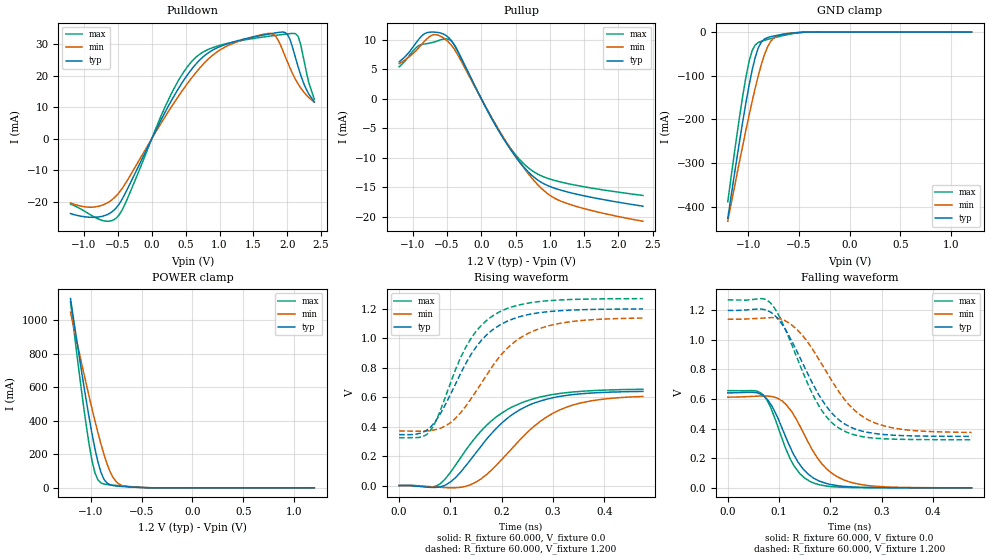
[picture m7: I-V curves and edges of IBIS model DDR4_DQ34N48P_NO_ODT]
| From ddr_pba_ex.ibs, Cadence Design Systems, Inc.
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|   Model DDR4_DQ34N48P_NO_ODT
[Model]   DDR4_DQ34N48P_NO_ODT
Model_type I/O
Polarity   Non-Inverting
Enable   Active-High
Vinl =  0.823V
Vinh =  0.887V
C_comp   1.689pF   1.691pF   1.711pF
C_comp_pullup   0.525pF   0.576pF   0.518pF
C_comp_pulldown   1.164pF   1.114pF   1.192pF
[Model Spec]
Vinh   0.887V   NA   NA
Vinl   0.823V   NA   NA
Vmeas   0.840V   NA   NA
[Temperature Range]   27.000   0.125k   -40.000
[Voltage Range]   1.200V   1.140V   1.270V
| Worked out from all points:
|   slope of the pulldown table from 0 to 0.18 V, typ, clamps not added: 23.3 ohm
|   slope of the pullup table from 0 to 0.18 V, typ, clamps not added: 45.9 ohm
|   GND clamp passes 1 mA (typ) near -0.50 V on its own axis
|   POWER clamp passes 1 mA (typ) near -0.46 V on its own axis
|   rising waveform, R_fixture 60.000, V_fixture 0.0: 20-80 % time 105ps typ, 111ps min, 106ps max; typ from 0.002 V to 0.64 V
|   rising waveform, R_fixture 60.000, V_fixture 1.200: 20-80 % time 87.2ps typ, 101ps min, 77.5ps max; typ from 0.346 V to 1.2 V
|   falling waveform, R_fixture 60.000, V_fixture 0.0: 20-80 % time 54.7ps typ, 65.3ps min, 47.2ps max; typ from 0.642 V to 0 V
|   falling waveform, R_fixture 60.000, V_fixture 1.200: 20-80 % time 80.4ps typ, 90.4ps min, 73.9ps max; typ from 1.2 V to 0.348 V
[Pulldown]
|Voltage   I(typ)   I(min)   I(max)
-1.2V     -23.72mA   -20.38mA   -20.68mA
-840mV    -24.88mA   -21.61mA   -24.88mA
-520mV    -21.78mA   -18mA      -25.05mA
400mV     16.1mA     13.66mA    18.67mA
640mV     23.35mA    20.64mA    25.58mA
960mV     28.73mA    27.44mA    29.28mA
1.76V     33.27mA    33.33mA    32.54mA
1.84V     33.56mA    32.14mA    32.76mA
2V        33.13mA    24.48mA    33.18mA
2.12V     25.82mA    18.86mA    33.28mA
2.2V      20.09mA    16.05mA    29.74mA
2.4V      11.64mA    11.56mA    12.48mA
[Pullup]
|Voltage   I(typ)   I(min)   I(max)
-1.2V     6.276mA    5.968mA    5.424mA
-960mV    9.396mA    8.108mA    8.597mA
-840mV    10.98mA    9.634mA    9.283mA
-720mV    11.33mA    10.8mA     9.54mA
-560mV    11.02mA    10.4mA     10.13mA
-400mV    9.244mA    8.51mA     9.292mA
280mV     -5.933mA   -5.721mA   -5.889mA
520mV     -10.14mA   -10.1mA    -9.786mA
760mV     -13.22mA   -13.77mA   -12.36mA
960mV     -14.69mA   -16.04mA   -13.47mA
1.2V      -15.64mA   -17.56mA   -14.24mA
2.36V     -18.24mA   -20.8mA    -16.42mA
[GND_clamp]
|Voltage   I(typ)   I(min)   I(max)
-1.2V     -426.2mA   -432.8mA   -388.3mA
-1.08V    -244.1mA   -290.9mA   -187.6mA
-1.02V    -160.2mA   -222.9mA   -101.2mA
-990mV    -121.8mA   -190.1mA   -66.76mA
-960mV    -87.12mA   -158.5mA   -42.47mA
-900mV    -36.37mA   -100.2mA   -23.99mA
-840mV    -16.17mA   -52.6mA    -18.98mA
-810mV    -12.75mA   -34.94mA   -17.06mA
-750mV    -9.219mA   -14.09mA   -13.42mA
-600mV    -3.476mA   -2.979mA   -5.372mA
-390mV    -77.95uA   -145.6uA   -88.64uA
1.2V      1.573nA    185.8nA    251.5pA
[POWER_clamp]
|Voltage   I(typ)   I(min)   I(max)
-1.2V     1.129A     1.047A     1.109A
-1.08V    651.1mA    713.3mA    524.8mA
-1.02V    430.1mA    553.1mA    270.8mA
-990mV    328mA      475.7mA    167mA
-960mV    234.7mA    400.6mA    90.32mA
-930mV    154.2mA    328.7mA    47.17mA
-900mV    91.53mA    260.8mA    29.3mA
-840mV    28.2mA     142.5mA    19.67mA
-780mV    13.3mA     60.49mA    15.94mA
-720mV    9.309mA    21.57mA    12.7mA
-660mV    6.902mA    8.818mA    9.642mA
1.2V      -4.11nA    -153.5nA   -872pA
[Ramp]
| variable   typ   min   max
dV/dt_r 0.348/0.102n   0.332/0.111n   0.351/0.102n
dV/dt_f 0.481/82.840p   0.430/93.487p   0.535/75.995p
R_load = 50.000
| The next line is not an IBIS keyword
| [Initial Delay]   0.325ns   0.500ns   0.200ns
[Rising Waveform]
R_fixture= 60.000
V_fixture= 0.0
V_fixture_min= 0.0
V_fixture_max= 0.0
|time   V(typ)   V(min)   V(max)
0s        1.745mV    1.208mV    364.9uV
66ps      -11.98mV   -7.582mV   -8.093mV
99ps      22.37mV    -14.41mV   85.62mV
158ps     262.2mV    42.12mV    365.4mV
203ps     434.6mV    189.1mV    499.9mV
238ps     520.7mV    321.3mV    561.8mV
285ps     584.6mV    461.1mV    609.5mV
326ps     612.8mV    532.8mV    631.4mV
386ps     631.1mV    582mV      646.6mV
475ps     639.7mV    605.5mV    654.3mV
[Rising Waveform]
R_fixture= 60.000
V_fixture= 1.200
V_fixture_min= 1.140
V_fixture_max= 1.270
|time   V(typ)   V(min)   V(max)
0s        346.5mV    371.3mV    325.1mV
58ps      388.6mV    372.9mV    361.5mV
73ps      448.3mV    382.4mV    448.5mV
98ps      605.5mV    421.9mV    679.6mV
129ps     824.2mV    535.4mV    935mV
158ps     977.3mV    684.2mV    1.08V
188ps     1.072V     841.4mV    1.165V
228ps     1.139V     984.2mV    1.221V
285ps     1.179V     1.079V     1.254V
475ps     1.199V     1.137V     1.27V
[Falling Waveform]
R_fixture= 60.000
V_fixture= 0.0
V_fixture_min= 0.0
V_fixture_max= 0.0
|time   V(typ)   V(min)   V(max)
0s        641.7mV    612.7mV    657mV
70ps      619.8mV    621.1mV    625.2mV
87ps      547.4mV    616.5mV    513mV
106ps     402.6mV    587.2mV    330.1mV
129ps     222mV      490mV      149.7mV
147ps     126.5mV    374.6mV    74.89mV
169ps     62.17mV    232.6mV    30.41mV
205ps     19.52mV    93.62mV    7.468mV
246ps     5.364mV    31.59mV    1.875mV
475ps     129.2uV    183.3uV    57.78uV
[Falling Waveform]
R_fixture= 60.000
V_fixture= 1.200
V_fixture_min= 1.140
V_fixture_max= 1.270
|time   V(typ)   V(min)   V(max)
0s        1.199V     1.139V     1.27V
65ps      1.209V     1.147V     1.279V
83ps      1.188V     1.15V      1.251V
105ps     1.11V      1.139V     1.127V
143ps     862.9mV    1.041V     808.4mV
179ps     619.8mV    859.7mV    544.6mV
223ps     442.9mV    618.4mV    390.2mV
256ps     388.8mV    498.1mV    350.1mV
304ps     360.4mV    419.2mV    331.5mV
475ps     347.6mV    374.6mV    325.1mV
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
